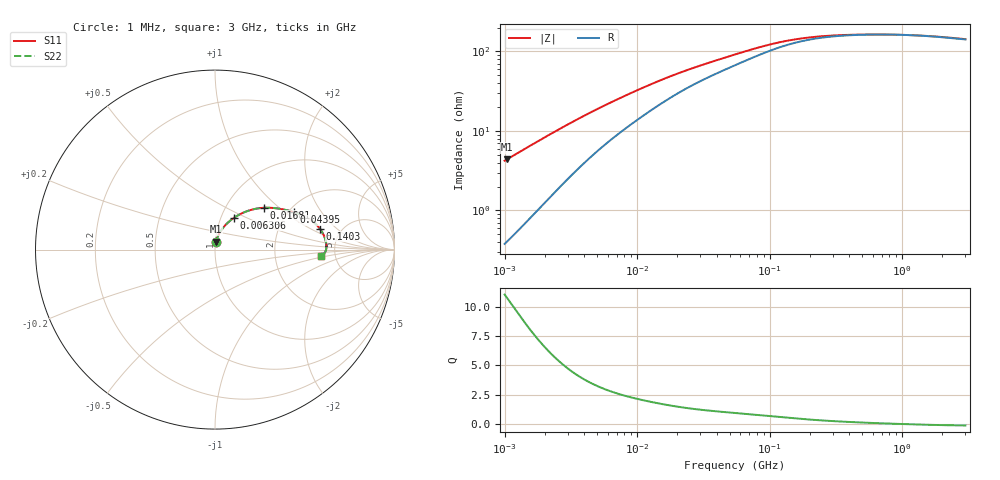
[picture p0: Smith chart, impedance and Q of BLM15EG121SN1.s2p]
! BLM15EG121SN1
# Hz S RI R 50
!Freq.(Hz) S11(Real) S11(Imag) S21(Real) S21(Imag) S12(Real) S12(Imag) S22(Real) S22(Imag)
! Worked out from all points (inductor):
!   401 points, 1 MHz to 3 GHz, reference 50 ohm
!   read as one part in series: L = 665 nH near 1.041 MHz
!   highest Q = 10.8 at 1.041 MHz (marker M1), where L = 669 nH
!   self-resonance near 916 MHz
!   S11 on the Smith chart (normalised r, x): 1 MHz: 1.01, +0.08; 6.306 MHz: 1.15, +0.43; 16.81 MHz: 1.49, +0.80; 43.95 MHz: 2.14, +1.17; 140.3 MHz: 3.46, +1.25; 3 GHz: 3.83, -0.39
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1000000  0.00553 0.0417  0.9945 -0.0417  0.9945 -0.0417  0.00553 0.0417
1040844  0.00592 0.0433  0.9941 -0.0433  0.9941 -0.0433  0.00592 0.0433
1522470  0.0115 0.0621  0.9885 -0.0621  0.9885 -0.0621  0.0115 0.0621
2182827  0.0218 0.0857  0.9782 -0.0857  0.9782 -0.0857  0.0218 0.0857
2947212  0.0361 0.1096  0.9639 -0.1096  0.9639 -0.1096  0.0361 0.1096
3823119  0.0543 0.1326  0.9457 -0.1326  0.9457 -0.1326  0.0543 0.1326
4861065  0.0766 0.1546  0.9234 -0.1546  0.9234 -0.1546  0.0766 0.1546
6305767  0.1069 0.1779  0.8931 -0.1779  0.8931 -0.1779  0.1069 0.1779
9600343  0.1692 0.2106  0.8308 -0.2106  0.8308 -0.2106  0.1692 0.2106
1.461624e7  0.2454 0.2305  0.7546 -0.2305  0.7546 -0.2305  0.2454 0.2305
1.681455e7  0.2723 0.233  0.7277 -0.233  0.7277 -0.233  0.2723 0.233
2.559965e7  0.3507 0.2289  0.6493 -0.2289  0.6493 -0.2289  0.3507 0.2289
4.394807e7  0.441 0.2084  0.559 -0.2084  0.559 -0.2084  0.441 0.2084
5.477226e7  0.4751 0.1964  0.5249 -0.1964  0.5249 -0.1964  0.4751 0.1964
9.034013e7  0.5431 0.1582  0.4569 -0.1582  0.4569 -0.1582  0.5431 0.1582
1.403209e8  0.5841 0.1168  0.4159 -0.1168  0.4159 -0.1168  0.5841 0.1168
2.094008e8  0.6052 0.0815  0.3948 -0.0815  0.3948 -0.0815  0.6052 0.0815
2.771263e8  0.6135 0.0605  0.3865 -0.0605  0.3865 -0.0605  0.6135 0.0605
3.817355e8  0.6186 0.0404  0.3814 -0.0404  0.3814 -0.0404  0.6186 0.0404
8.005644e8  0.62 0.00533  0.38 -0.00533  0.38 -0.00533  0.62 0.00533
1.488926e9  0.6115 -0.0174  0.3885 0.0174  0.3885 0.0174  0.6115 -0.0174
3e9  0.5888 -0.033  0.4112 0.033  0.4112 0.033  0.5888 -0.033
